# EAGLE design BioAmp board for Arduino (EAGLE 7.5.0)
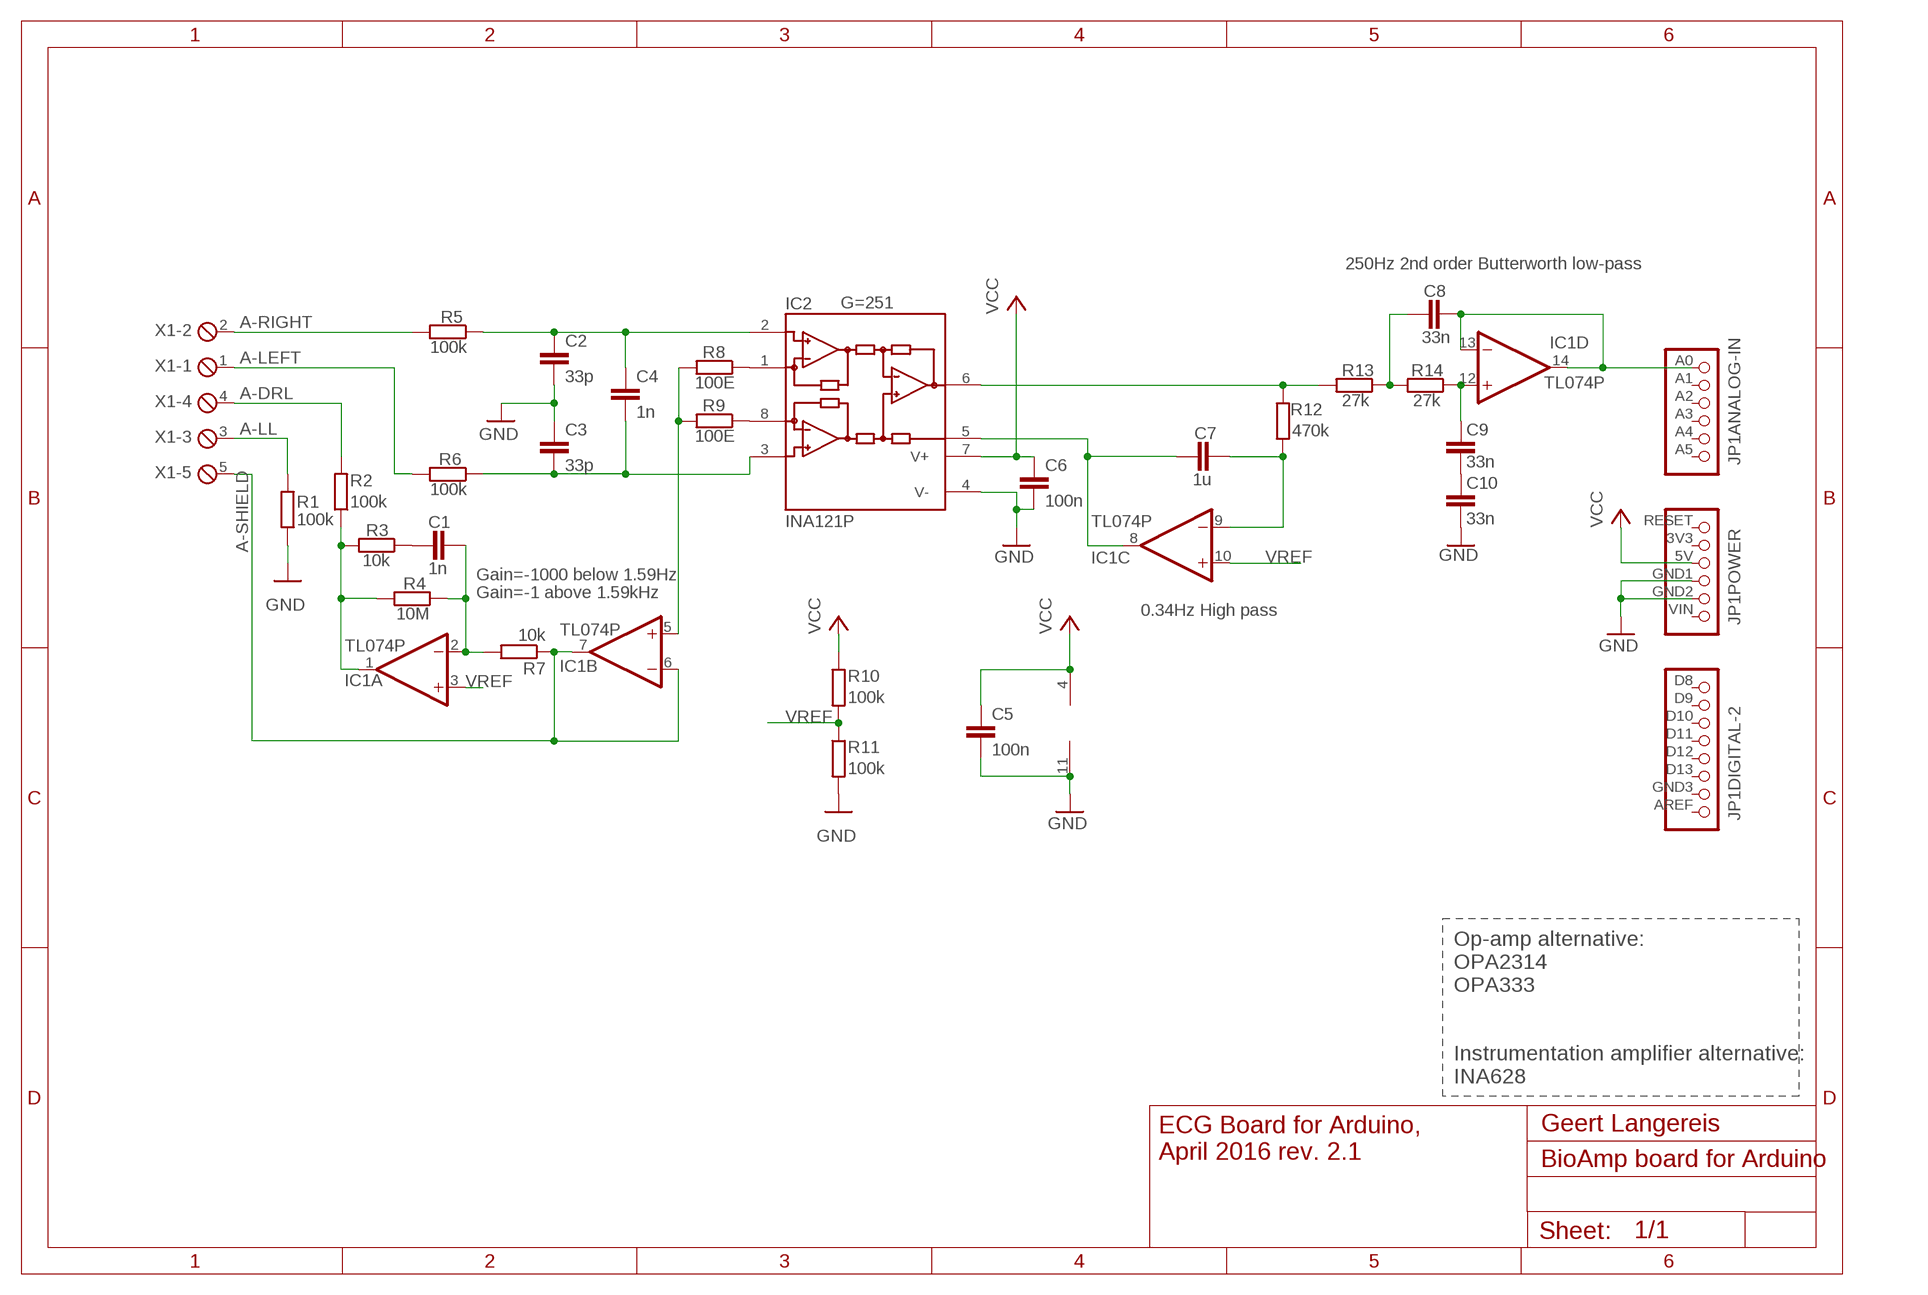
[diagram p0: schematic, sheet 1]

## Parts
C1  1n  C2.5/2  [C2.5-2]
C2  33p  C2.5/2  [C2.5-2]
C3  33p  C2.5/2  [C2.5-2]
C4  1n  C2.5/2  [C2.5-2]
C5  100n  C5/2.5  [C5B2.5]
C6  100n  C5/2.5  [C5B2.5]
C7  1u  C5/3  [C5B3]
C8  33n  C2.5/2  [C2.5-2]
C9  33n  C2.5/2  [C2.5-2]
C10  33n  C2.5/2  [C2.5-2]
IC1  TL074P  [DIL14]
IC2  INA121P  [DIL08]
JP1  ARDUINO-2009"  [ARDUINO-HEADER]
R1  100k  R-EU_0204/7  [0204/7]
R2  100k  R-EU_0204/7  [0204/7]
R3  10k  R-EU_0204/7  [0204/7]
R4  10M  R-EU_0204/7  [0204/7]
R5  100k  R-EU_0204/7  [0204/7]
R6  100k  R-EU_0204/7  [0204/7]
R7  10k  R-EU_0204/7  [0204/7]
R8  100E  R-EU_0204/7  [0204/7]
R9  100E  R-EU_0204/7  [0204/7]
R10  100k  R-EU_0204/7  [0204/7]
R11  100k  R-EU_0204/7  [0204/7]
R12  470k  R-EU_0204/7  [0204/7]
R13  27k  R-EU_0204/7  [0204/7]
R14  27k  R-EU_0204/7  [0204/7]
X1  MPT5  [5POL254]

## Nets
A-DRL: R2.2 X1.4
A-LEFT: R6.2 X1.1
A-LL: R1.2 X1.3
A-RIGHT: R5.2 X1.2
A-SHIELD: IC1.6(B:-IN) IC1.7(B:OUT) R7.1 X1.5
GND: C2.2 C3.1 C5.2 C6.2 C10.1 IC1.11(P:V-) IC2.4(V-) JP1.GND1 JP1.GND2 R1.1 R11.2
N$1: IC1.1(A:OUT) R2.1 R3.2 R4.2
N$2: IC2.1(RG) R8.1
N$3: IC2.8(RG) R9.1
N$4: IC1.5(B:+IN) R8.2 R9.2
N$5: IC2.6(OUT) R12.1 R13.2
N$6: C8.1 R13.1 R14.2
N$8: C9.2 IC1.12(D:+IN) R14.1
N$9: C1.2 IC1.2(A:-IN) R4.1 R7.2
N$10: C9.1 C10.2
N$12: C8.2 IC1.13(D:-IN) IC1.14(D:OUT) JP1.A0
N$13: C7.1 IC1.9(C:-IN) R12.2
N$16: C7.2 IC1.8(C:OUT) IC2.5(REF)
N$17: C1.1 R3.1
N$22: C2.1 C4.1 IC2.2(-IN) R5.1
N$23: C3.2 C4.2 IC2.3(+IN) R6.1
VCC: C5.1 C6.1 IC1.4(P:V+) IC2.7(V+) JP1.5V R10.1
VREF: IC1.3(A:+IN) IC1.10(C:+IN) R10.2 R11.1
Unconnected: JP1.3V3 JP1.A1 JP1.A2 JP1.A3 JP1.A4 JP1.A5 JP1.AREF JP1.D0 JP1.D1 JP1.D2 JP1.D3 JP1.D4 JP1.D5 JP1.D6 JP1.D7 JP1.D8 JP1.D9 JP1.D10 JP1.D11 JP1.D12 JP1.D13 JP1.GND3 JP1.RESET JP1.VIN

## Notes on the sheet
- 250Hz 2nd order Butterworth low-pass
- G=251
- Gain=-1000 below 1.59Hz
- Gain=-1 above 1.59kHz
- 0.34Hz High pass
- Op-amp alternative:
  OPA2314
  OPA333
  
  
  Instrumentation amplifier alternative:
  INA628
- Geert Langereis
- ECG Board for Arduino,
  April 2016 rev. 2.1

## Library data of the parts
C1-C10 = capacitor-wima:C: CAPACITOR
IC1 = linear:TL074: OP AMP
IC2 = Geert-library:INA121: Instrumentation Amplifiers FET Input, Low Power
JP1 = zelf:ARDUINO-2009: Arduino board Arduino Duemilanove
R1-R14 = rcl:R-EU_: RESISTOR, European symbol
X1 = con-phoenix-254:MPT5: PHOENIX CONNECTOR; OC_FARNELL: unknown; OC_NEWARK: unknown

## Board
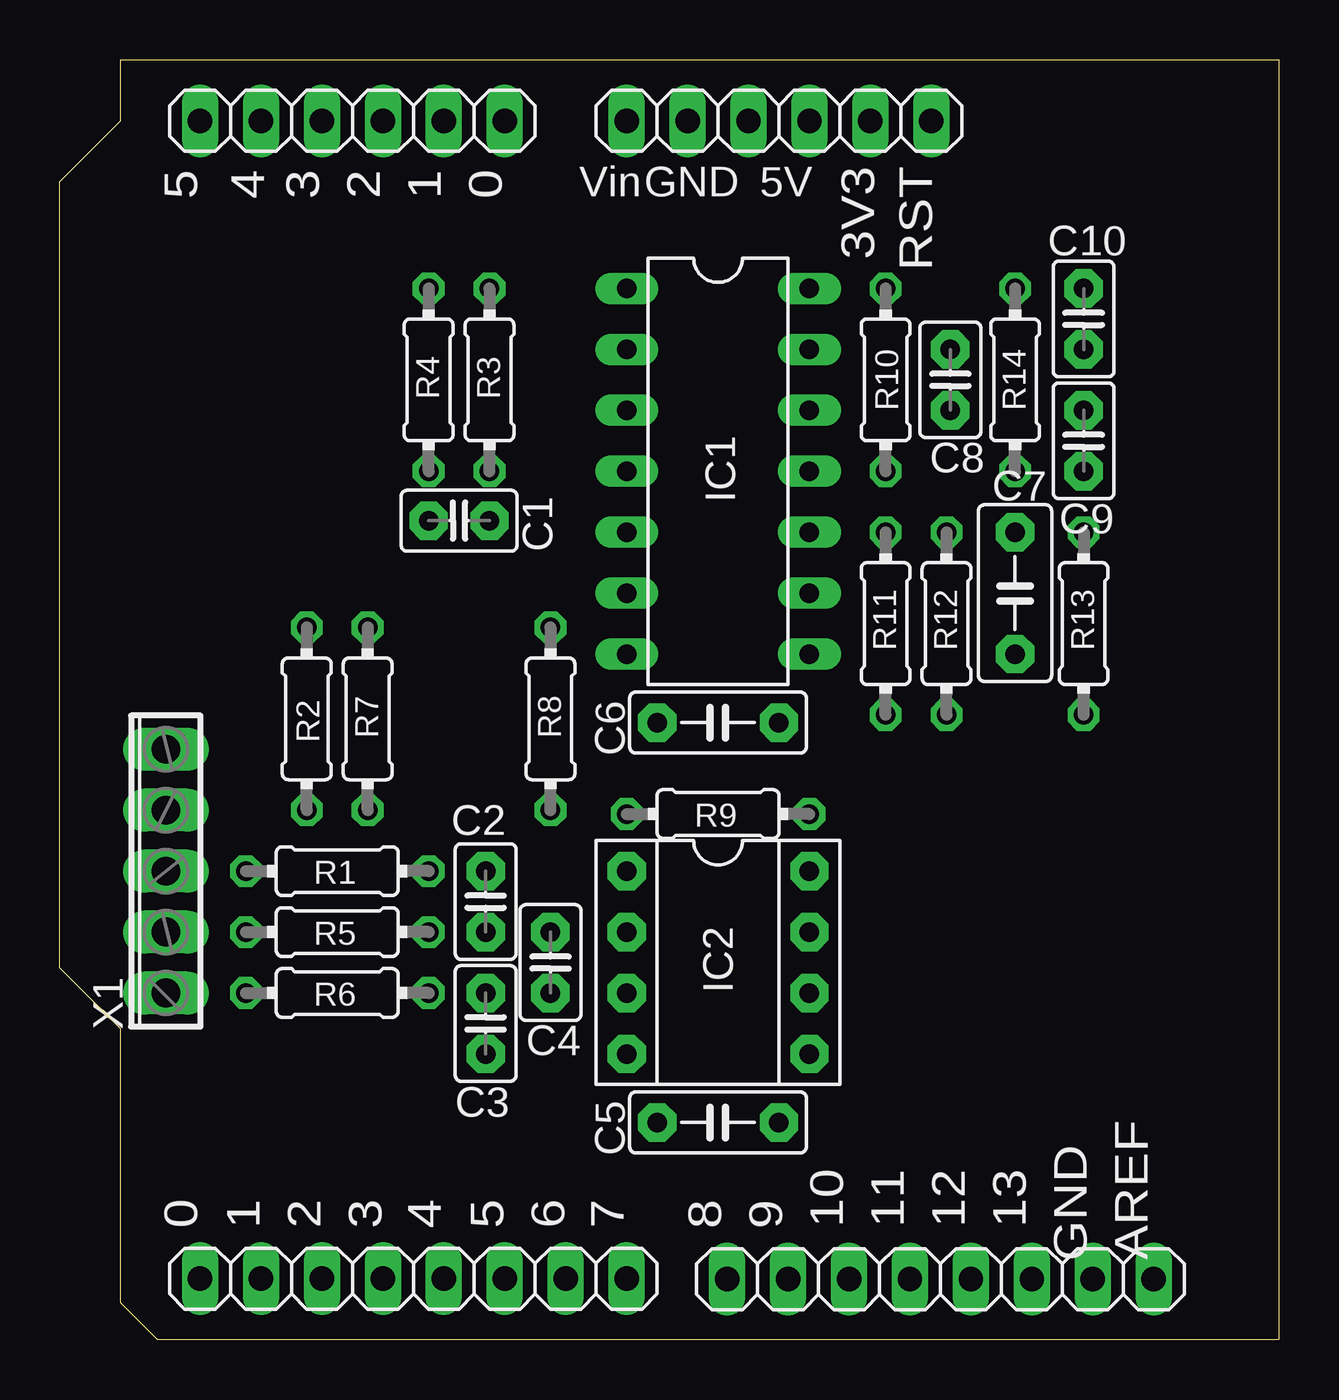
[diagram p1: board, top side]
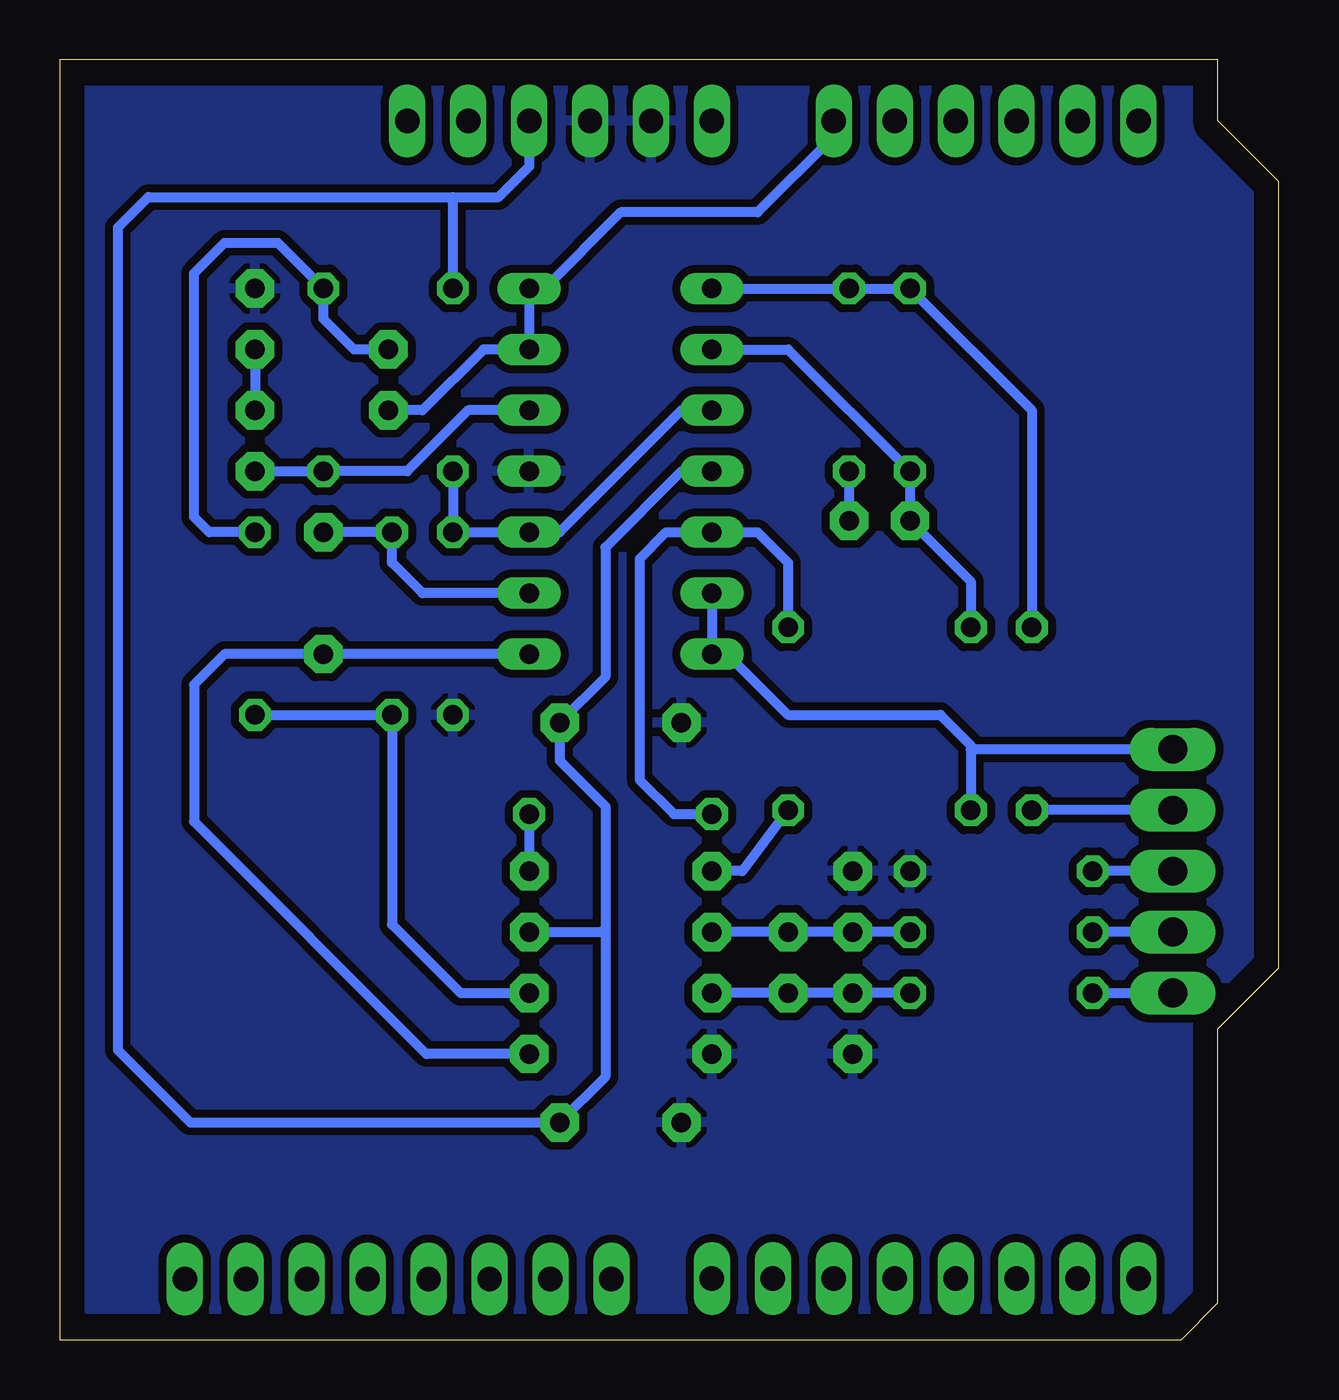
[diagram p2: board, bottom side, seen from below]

Size 50.8 x 53.34 mm. Coordinates in mm from the lower left corner, seen from the top.
Outline: 50.8,0 4.06,0 2.54,1.52 2.54,12.95 0,15.49 0,48.26 2.54,50.8 2.54,53.34 50.8,53.34 50.8,0
Copper layers (1*16): Top 0.035mm / dielectric 1.5mm / Bottom 0.035mm
Design rules "default *": minimum track width 10mil, minimum drill 24mil, track to track 13mil, track to pad 13mil, pad to pad 13mil, via to via 13mil, smd to smd 8mil, copper to edge 40mil, drill to drill 8mil, minimum pad ring 10mil, minimum via ring 8mil, stop-mask expansion 4mil, vias tented up to drill 0mil, thermal gap 10mil

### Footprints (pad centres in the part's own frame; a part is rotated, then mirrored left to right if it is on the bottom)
C2.5-2 = drill 0.813 pad 1.6 octagon: 1 -1.27,0; 2 1.27,0
C5B2.5 = drill 0.813 pad 1.6 octagon: 1 -2.54,0; 2 2.54,0
C5B3 = drill 0.813 pad 1.6 octagon: 1 -2.54,0; 2 2.54,0
DIL14 = drill 0.813 long: 1 -7.62,-3.81; 2 -5.08,-3.81; 3 -2.54,-3.81; 4 0,-3.81; 5 2.54,-3.81; 6 5.08,-3.81; 7 7.62,-3.81; 8 7.62,3.81; 9 5.08,3.81; 10 2.54,3.81; 11 0,3.81; 12 -2.54,3.81; 13 -5.08,3.81; 14 -7.62,3.81
DIL08 = drill 0.813 pad 1.6 octagon: 1 -3.81,-3.81; 2 -1.27,-3.81; 3 1.27,-3.81; 4 3.81,-3.81; 5 3.81,3.81; 6 1.27,3.81; 7 -1.27,3.81; 8 -3.81,3.81
ARDUINO-HEADER = drill 1.016 long: 3V3 2.54,-48.26; 5V 5.08,-48.26; A0 17.78,-48.26; A1 20.32,-48.26; A2 22.86,-48.26; A3 25.4,-48.26; A4 27.94,-48.26; A5 30.48,-48.26; AREF -9.271,0.025; D0 30.48,0; D1 27.94,0; D2 25.4,0; D3 22.86,0; D4 20.32,0; D5 17.78,0; D6 15.24,0; D7 12.7,0; D8 8.509,0.025; D9 5.969,0.025; D10 3.429,0.025; D11 0.889,0.025; D12 -1.651,0.025; D13 -4.191,0.025; GND1 7.62,-48.26; GND2 10.16,-48.26; GND3 -6.731,0.025; RESET 0,-48.26; VIN 12.7,-48.26
0204/7 = drill 0.813 octagon: 1 -3.81,0; 2 3.81,0
5POL254 = drill 1.2 long: 1 -5.08,0; 2 -2.54,0; 3 0,0; 4 2.54,0; 5 5.08,0

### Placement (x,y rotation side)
C1  16.64,34.13 180 top
C2  17.75,18.26 90 top
C3  17.75,13.18 90 top
C4  20.45,15.72 270 top
C5  27.43,9.05 180 top
C6  27.43,25.72 180 top
C7  39.81,31.11 270 top
C8  37.12,40 270 top
C9  42.67,37.47 270 top
C10  42.67,42.55 270 top
DRILEGEND  [DRILEGEND]  not placed on the board
IC1  27.43,36.2 270 top
IC2  27.43,15.72 270 top
JP1  36.32,2.54 180 top
R1  11.56,19.53 180 top
R2  10.29,25.88 270 top
R3  17.91,40 90 top
R4  15.37,40 90 top
R5  11.56,16.99 180 top
R6  11.56,14.45 180 top
R7  12.83,25.88 90 top
R8  20.45,25.88 90 top
R9  27.43,21.91 180 top
R10  34.42,40 270 top
R11  34.42,29.84 270 top
R12  36.96,29.84 90 top
R13  42.67,29.84 270 top
R14  39.81,40 90 top
X1  4.41,19.53 90 top

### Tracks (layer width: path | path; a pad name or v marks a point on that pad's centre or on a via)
A-DRL
  Bottom 0.406: X1.4 R2.2
A-LEFT
  Bottom 0.406: R6.2 X1.1
A-LL
  Bottom 0.406: X1.3 R1.2
A-RIGHT
  Bottom 0.406: X1.2 R5.2
A-SHIELD
  Bottom 0.406: X1.5 12.83,24.61 | IC1.6 IC1.7 22.99,28.57 20.45,26.03 14.1,26.03 12.83,24.77 12.83,24.61 | 12.83,24.61 R7.1
GND
  pour Bottom: 3.3,2.54 4.57,1.27 49.66,1.27 50.29,52.07 3.3,52.07 3.3,50.16 0.76,47.62 0.76,15.88 3.3,13.34
N$1
  Bottom 0.406: IC1.1 R3.2 R4.2 10.29,38.73 R2.1
N$2
  Bottom 0.406: R8.1 22.35,19.53 IC2.1
N$3
  Bottom 0.406: R9.1 IC2.8
N$4
  Bottom 0.406: IC1.5 24.42,33.66 | R9.2 25.21,21.91 26.64,23.34 26.64,32.54 25.53,33.66 IC1.5 | IC1.5 21.72,33.66 20.45,32.38 R8.2
N$5
  Bottom 0.406: R13.2 R12.1 36.96,17.3 34.1,14.45 IC2.6
N$6
  Bottom 0.406: C8.1 38.55,41.27 39.81,42.55 R14.2 41.72,45.72 43.94,45.72 45.21,44.45 45.21,34.29 44.58,33.66 R13.1
N$8
  Bottom 0.406: C9.2 R14.1 36.32,36.2 33.78,38.73 IC1.12
N$9
  Bottom 0.406: IC1.2 20.45,41.27 R4.1 C1.2 12.83,31.59 R7.2
N$10
  Bottom 0.406: C10.2 C9.1
N$12
  Bottom 0.406: C8.2 35.69,38.73 33.15,41.27 IC1.13 IC1.14 30.61,43.81 27.43,46.99 21.72,46.99 18.54,50.16 JP1.A0
N$13
  Bottom 0.406: C7.1 R12.2 36.96,32.38 35.69,31.11 IC1.9
N$16
  Bottom 0.406: IC1.8 C7.2 43.94,28.57 45.21,27.3 45.21,21.59 35.53,11.91 IC2.5
N$17
  Bottom 0.406: R3.1 C1.1
N$22
  Bottom 0.406: R5.1 C2.1 C4.1 IC2.2
N$23
  Bottom 0.406: R6.1 C3.2 C4.2 IC2.3
VCC
  Bottom 0.406: C5.1 45.37,9.05 48.39,12.06 48.39,46.36 47.12,47.62 34.42,47.62 | C5.1 29.81,9.05 | IC1.4 24.89,36.2 28.07,33.02 28.07,27.62 C6.1 29.97,24.13 28.07,22.23 28.07,17.14 | 28.07,17.14 28.07,10.95 C5.1 | IC2.7 28.23,16.99 28.07,17.14 | JP1.5V 31.24,48.89 32.51,47.62 34.42,47.62 | R10.1 34.42,47.62
VREF
  Bottom 0.406: R10.2 R11.1 IC1.10 29.97,33.66 24.89,38.73 IC1.3

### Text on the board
tNames: Vin | GND | 5V | 3V3 | RST | 5 | 4 | 3 | 2 | 1 | 0 | AREF | GND | 10 | 11 | 12 | 13 | 0 | 1 | 2 | 3 | 4 | 5 | 6 | 7 | 8 | 9
tValues: GND | +5V | SH | LL | DRL | RA | LA | Fontys 2016
ArduinoHoles: 3.2mm | 2.2mm | 3.2mm
DrillLegend: LAYER-STACK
